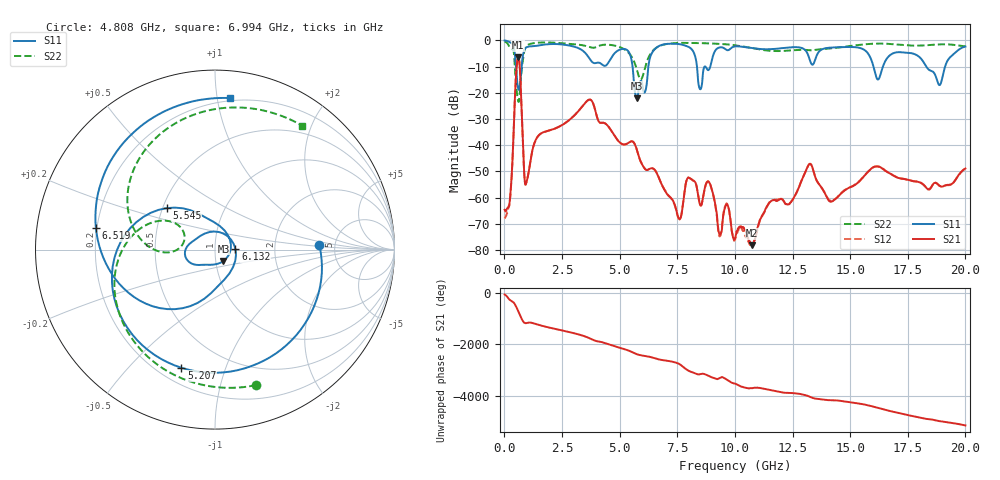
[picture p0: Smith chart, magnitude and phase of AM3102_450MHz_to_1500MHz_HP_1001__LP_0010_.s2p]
!Agilent Technologies,E8364B,MY43040894,A.07.50.67
!Agilent E8364B: A.07.50.67
!Date: Thursday, January 11, 2018 06:01:22
!Correction: S11(Full 2 Port(1,2))
!S21(Full 2 Port(1,2))
!S12(Full 2 Port(1,2))
!S22(Full 2 Port(1,2))
!S2P File: Measurements: S11, S21, S12, S22:
# Hz S  dB  R 50
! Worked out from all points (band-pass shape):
!   1601 points, 10 MHz to 20 GHz, reference 50 ohm
!   highest |S21| = -6.48 dB at 597.2 MHz (marker M1); lowest = -78.2 dB at 10.75 GHz (marker M2)
!   |S21| within 3 dB of the highest: 540.5 MHz to 662.2 MHz (121.7 MHz wide, 20.2 % of centre)
!   lowest |S11| = -22.0 dB at 5.745 GHz (marker M3), VSWR 1.17, Z = 54.5 - j6.97 ohm
!   |S11| at or under -10 dB: 5.56 GHz to 6.246 GHz (685.7 MHz wide, 11.6 % of centre); 16.01 GHz to 16.42 GHz (411.2 MHz wide, 2.54 % of centre); 18.3 GHz to 19.12 GHz (815.9 MHz wide, 4.36 % of centre)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
!   |S22| runs from -23.5 to -0.4 dB; largest |S21 - S12| = 0.00088
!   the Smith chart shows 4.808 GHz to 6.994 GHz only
!   S11 on the Smith chart (normalised r, x): 4.808 GHz: 3.77, +0.26; 5.207 GHz: 0.29, -0.71; 5.545 GHz: 0.52, +0.28; 6.132 GHz: 1.26, +0.01; 6.519 GHz: 0.20, +0.09; 6.994 GHz: 0.18, +1.09
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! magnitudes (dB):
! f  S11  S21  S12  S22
! 10 MHz  0.0  -64.6  -67.9  -0.4
! 259.9 MHz  -0.8  -58.5  -59.0  -3.0
! 597.2 MHz  -18.4  -6.5  -6.5  -23.1
! 959.5 MHz  -2.7  -54.1  -54.0  -2.1
! 1.459 GHz  -2.0  -36.5  -36.6  -0.9
! 3.346 GHz  -3.6  -25.5  -25.5  -1.8
! 4.808 GHz  -4.7  -36.8  -36.8  -2.1
! 5.207 GHz  -3.3  -39.7  -39.7  -3.5
! 5.545 GHz  -9.0  -38.5  -38.5  -6.6
! 5.745 GHz  -22.0  -41.6  -41.6  -11.1
! 6.132 GHz  -18.9  -49.3  -49.3  -9.5
! 6.519 GHz  -3.4  -49.4  -49.4  -3.3
! 6.682 GHz  -2.3  -51.9  -52.0  -2.4
! 6.994 GHz  -1.4  -57.8  -57.5  -1.5
! 8.493 GHz  -18.7  -62.7  -62.7  -1.1
! 10.01 GHz  -2.3  -75.6  -76.1  -1.9
! 10.75 GHz  -3.0  -78.2  -78.0  -3.0
! 13.34 GHz  -9.2  -48.0  -48.0  -3.8
! 14.17 GHz  -2.8  -61.6  -61.2  -3.1
! 16.68 GHz  -6.1  -50.5  -50.5  -1.3
! 18.88 GHz  -17.1  -55.5  -55.5  -1.5
! 20 GHz  -2.4  -48.9  -48.9  -2.3
